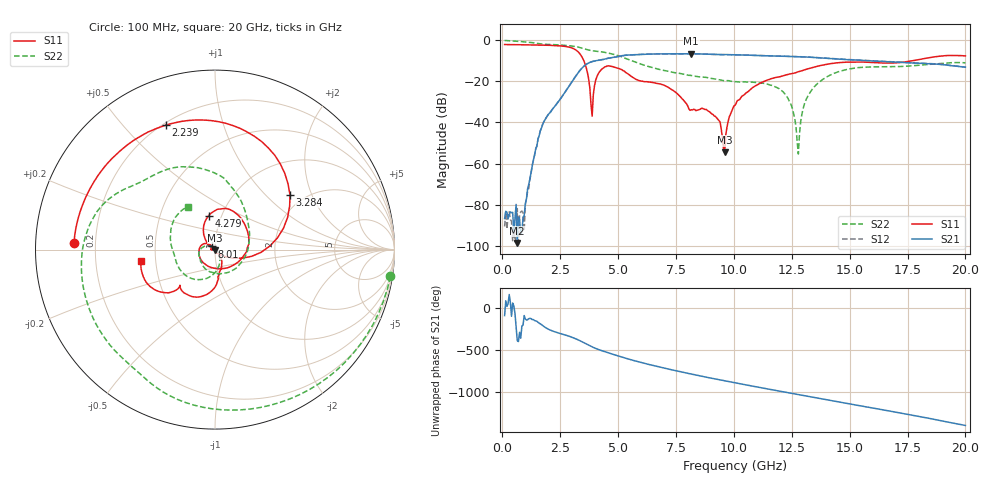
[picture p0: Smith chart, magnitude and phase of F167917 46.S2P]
!  2-Port S-parameters saved by WinCal
! VAR MeasName=S-Parameters (CALIBRATED_DATA) read from VNA (N5242A)
! VAR MeasDate=2016-11-22 9:02:04
! VAR NAME=F167917 46
! VAR FILENAME=F167917 46.S2P
! VAR DATE=2016-11-22 9:02:04
! VAR PHYS_PORTS=1,2
# Hz S DB R 50
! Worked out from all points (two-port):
!   401 points, 100 MHz to 20 GHz, reference 50 ohm
!   highest |S21| = -6.55 dB at 8.159 GHz (marker M1); lowest = -98.7 dB at 647.2 MHz (marker M2)
!   |S21| within 3 dB of the highest: 4.261 GHz to 15.12 GHz (10.86 GHz wide, 112 % of centre); 15.15599 GHz to 15.17881 GHz (22.82 MHz wide, 0.15 % of centre)
!   lowest |S11| = -54.6 dB at 9.602 GHz (marker M3), VSWR 1.00, Z = 50.1 - j0.16 ohm
!   |S11| at or under -10 dB: 3.522 GHz to 17.7 GHz (14.18 GHz wide, 134 % of centre)
!   |S22| runs from -55.4 to -0.1 dB; largest |S21 - S12| = 0.0066
!   S11 on the Smith chart (normalised r, x): 100 MHz: 0.12, +0.02; 2.239 GHz: 0.21, +0.66; 3.284 GHz: 1.69, +1.42; 4.279 GHz: 0.87, +0.34; 8.01 GHz: 0.96, +0.03; 20 GHz: 0.41, -0.06
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1e8  -2.09 177.3  -86.75 -88.0  -90.62 -162.0  -0.10 -8.7
6.4725e8  -2.16 162.8  -98.67 -27.5  -81.89 139.0  -0.49 -52.2
9.955e8  -2.22 153.3  -79.52 -127.7  -79.95 -134.8  -0.82 -77.5
1.64225e9  -2.35 133.9  -44.08 173.9  -44.05 174.1  -1.75 -118.3
2.23925e9  -2.55 111.5  -32.55 81.8  -32.55 81.4  -2.14 -147.9
3.284e9  -5.71 36.2  -15.72 -17.9  -15.74 -17.8  -3.34 159.8
3.43325e9  -7.97 17.3  -13.64 -38.5  -13.64 -38.4  -3.81 152.6
3.881e9  -36.95 171.8  -10.40 -101.0  -10.35 -101.0  -5.10 136.8
4.279e9  -14.29 100.4  -9.51 -144.3  -9.49 -144.5  -5.63 122.0
5.62225e9  -17.95 -50.3  -7.09 101.1  -7.07 101.0  -10.10 63.2
6.7665e9  -21.13 178.4  -6.64 20.9  -6.65 20.8  -14.17 13.7
8.01025e9  -32.00 135.5  -6.58 -55.3  -6.58 -55.3  -16.91 -65.7
8.1595e9  -33.80 158.0  -6.55 -64.2  -6.56 -64.4  -17.16 -74.3
9.1545e9  -36.89 -176.7  -6.92 -120.7  -6.91 -120.8  -18.80 -124.1
9.60225e9  -54.55 -58.5  -6.97 -144.3  -6.99 -144.2  -19.64 -136.2
1.005e10  -31.64 -48.9  -7.07 -168.6  -7.09 -168.5  -20.18 -145.9
1.204e10  -17.58 -79.2  -7.76 88.9  -7.71 88.8  -24.27 162.0
1.278625e10  -15.32 -84.9  -8.03 50.6  -7.99 50.8  -55.38 -24.8
1.338325e10  -13.30 -91.4  -8.32 19.7  -8.27 20.0  -23.94 -65.0
1.517425e10  -10.62 -122.4  -9.54 -68.8  -9.50 -68.9  -13.61 -130.2
1.67165e10  -11.09 -134.5  -10.43 -144.8  -10.42 -145.0  -12.88 -166.6
2e10  -7.61 -171.4  -13.11 42.9  -13.05 42.2  -11.00 122.5
